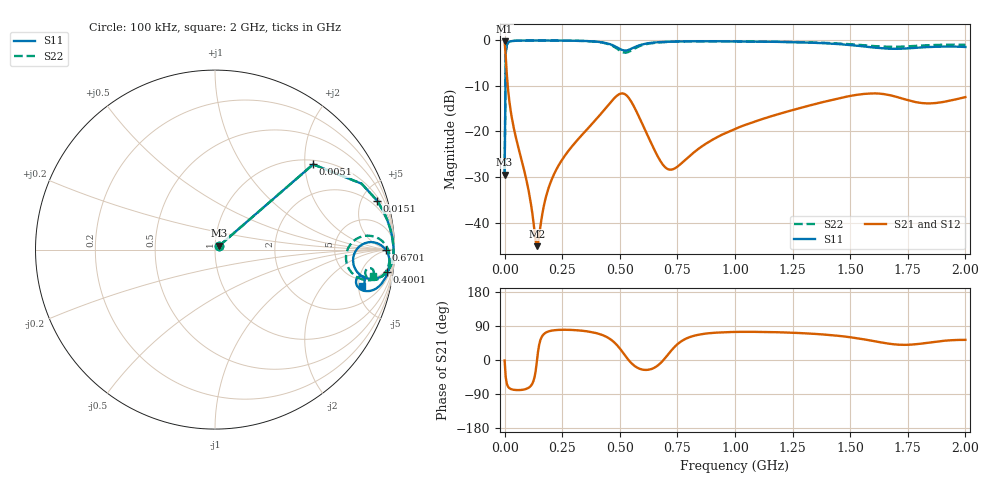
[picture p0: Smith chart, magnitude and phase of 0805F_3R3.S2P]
! Network Analyzer HP8753ES.07.68: Mar 08, 2001 Serial No. US39171556
! 21 Feb 2006  11:51:48
! Frequency  S11  S21  S12  S22
# HZ  S  RI R  50
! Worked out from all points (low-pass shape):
!   401 points, 100 kHz to 2 GHz, reference 50 ohm
!   highest |S21| = -0.21 dB at 100 kHz (marker M1); lowest = -45.2 dB at 140.1 MHz (marker M2)
!   |S21| within 3 dB of the highest: start of sweep to 4.486 MHz
!   lowest |S11| = -29.5 dB at 100 kHz (marker M3), VSWR 1.07, Z = 52.5 + j2.36 ohm
!   |S11| at or under -10 dB: start of sweep to 3.751 MHz
!   |S22| runs from -29.5 to 0.0 dB; largest |S21 - S12| = 0.0012
!   S11 on the Smith chart (normalised r, x): 100 kHz: 1.05, +0.05; 5.1 MHz: 1.10, +2.20; 15.1 MHz: 1.30, +6.52; 400.1 MHz: 4, -14; 670.1 MHz: 41, -3; 2 GHz: 3.84, -5.47
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100000  0.0249 0.0225  0.9754 -0.0211  0.9761 -0.0219  0.0249 0.0222
5099750  0.5465 0.4748  0.4546 -0.4758  0.4541 -0.4752  0.5469 0.4748
1.509925e7  0.9038 0.2727  0.0967 -0.2732  0.0966 -0.2727  0.9034 0.2725
2.509875e7  0.9566 0.1721  0.0431 -0.1723  0.0432 -0.1722  0.957 0.1718
4.509775e7  0.982 0.0933  0.018 -0.0932  0.0181 -0.093  0.9819 0.0933
1.00095e8  0.9935 0.0242  0.00674 -0.0245  0.00674 -0.0244  0.9934 0.0257
1.40093e8  0.9946 0.000518  0.00551 -0.00036  0.00552 -0.000368  0.9947 0.00247
1.500925e8  0.9949 -0.00482  0.0055 0.00464  0.00548 0.00466  0.9946 -0.00293
1.80091e8  0.9941 -0.0182  0.00578 0.0185  0.00577 0.0185  0.9941 -0.0171
2.100895e8  0.9932 -0.0317  0.00666 0.0314  0.00665 0.0314  0.9935 -0.0299
3.350832e8  0.9806 -0.0876  0.02 0.0889  0.02 0.0889  0.9794 -0.0866
4.0008e8  0.9557 -0.1269  0.0459 0.1304  0.0459 0.1305  0.9518 -0.129
4.750762e8  0.8531 -0.1612  0.1568 0.1686  0.1566 0.1686  0.8323 -0.1685
5.250738e8  0.7701 -0.0469  0.2494 0.0447  0.2492 0.0448  0.7301 -0.0338
5.750712e8  0.8618 0.0413  0.1506 -0.0547  0.1505 -0.0547  0.8355 0.0764
6.700665e8  0.9532 -0.00385  0.0493 -0.0105  0.0492 -0.0104  0.9456 0.033
7.350632e8  0.9673 -0.0345  0.0327 0.0211  0.0327 0.0211  0.9636 0.00125
1.00005e9  0.9653 -0.1166  0.0292 0.1026  0.0292 0.1027  0.97 -0.075
1.335033e9  0.9175 -0.2013  0.069 0.1833  0.0688 0.1833  0.9357 -0.1449
1.670016e9  0.7855 -0.1825  0.1836 0.1705  0.1831 0.1713  0.8372 -0.131
1.835008e9  0.8272 -0.1538  0.1425 0.1448  0.1422 0.1455  0.8752 -0.1068
2e9  0.8185 -0.2052  0.1429 0.1903  0.1423 0.1908  0.878 -0.1454
